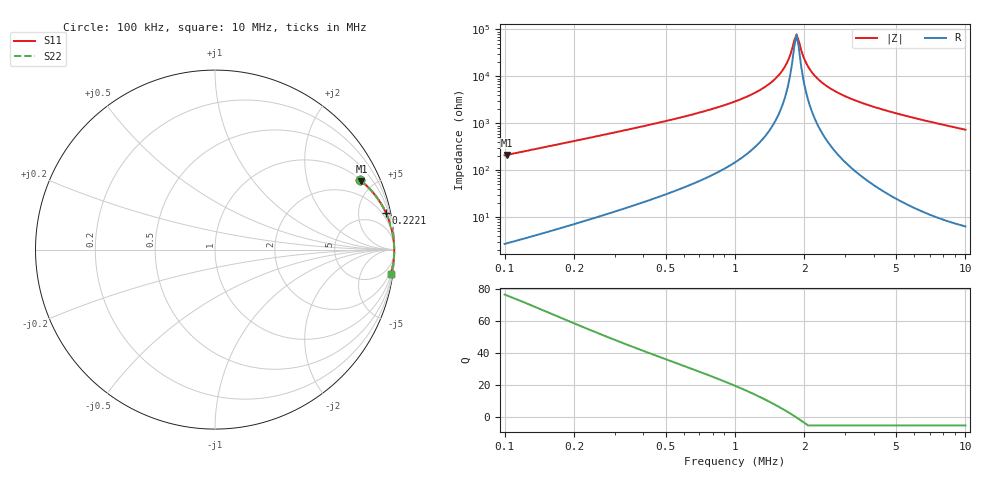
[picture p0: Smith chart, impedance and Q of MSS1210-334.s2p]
# MHz S MA R 50
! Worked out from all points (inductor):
!   203 points, 100 kHz to 10 MHz, reference 50 ohm
!   read as one part in series: L = 330 uH near 102.3 kHz
!   highest Q = 76.2 at 102.3 kHz (marker M1), where L = 331 uH
!   self-resonance near 1.809 MHz
!   S11 on the Smith chart (normalised r, x): 100 kHz: 1.05, +4.16; 222.1 kHz: 1.17, +9.34; 10 MHz: 1, -15
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0.1  0.8967 25.5  0.4312 -63.7  0.4312 -63.7  0.8967 25.5
0.102306  0.9005 25.0  0.4232 -64.2  0.4232 -64.2  0.9005 25.0
0.1507363  0.9489 17.6  0.3017 -71.6  0.3017 -71.6  0.9489 17.6
0.2220929  0.9743 12.0  0.2086 -76.9  0.2086 -76.9  0.9743 12.0
0.3424944  0.988 7.7  0.1344 -81.0  0.1344 -81.0  0.988 7.7
0.5046268  0.9937 5.0  0.08799 -83.4  0.08799 -83.4  0.9937 5.0
1.200074  0.9982 1.3  0.02328 -84.8  0.02328 -84.8  0.9982 1.3
1.440177  0.9985 0.8  0.01323 -83.0  0.01323 -83.0  0.9985 0.8
1.651284  0.9986 0.3  0.006046 -76.8  0.006046 -76.8  0.9986 0.3
1.768173  0.9987 0.1  0.002657 -60.4  0.002657 -60.4  0.9987 0.1
1.808947  0.9987 0.1  0.001712 -41.0  0.001712 -41.0  0.9987 0.1
1.85066  0.9987 -0.0  0.00128 2.9  0.00128 2.9  0.9987 -0.0
1.936996  0.9987 -0.1  0.002748 62.8  0.002748 62.8  0.9987 -0.1
2.027359  0.9988 -0.3  0.004985 75.5  0.004985 75.5  0.9988 -0.3
2.121938  0.9988 -0.4  0.007326 80.1  0.007326 80.1  0.9988 -0.4
2.272143  0.9988 -0.6  0.01091 83.2  0.01091 83.2  0.9988 -0.6
2.726739  0.9987 -1.2  0.02083 85.8  0.02083 85.8  0.9987 -1.2
3.424944  0.9984 -2.0  0.03427 86.4  0.03427 86.4  0.9984 -2.0
5.162633  0.9971 -3.6  0.06344 85.5  0.06344 85.5  0.9971 -3.6
6.787083  0.9951 -5.1  0.0884 84.3  0.0884 84.3  0.9951 -5.1
8.524974  0.9924 -6.5  0.114 82.9  0.114 82.9  0.9924 -6.5
10  0.9896 -7.8  0.1351 81.7  0.1351 81.7  0.9896 -7.8
